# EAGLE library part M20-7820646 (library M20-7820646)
M20: 6 Pos Receptacle SIL Straight 3mm THT Connector 8.5mm high Tin Source: Datasheet
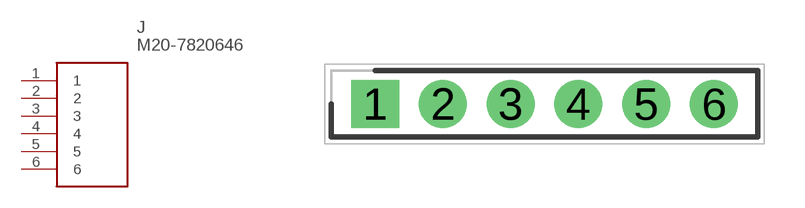
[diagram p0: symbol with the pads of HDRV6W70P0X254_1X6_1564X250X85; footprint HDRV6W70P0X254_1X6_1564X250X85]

Designator prefix J

## M20-7820646 (Description: M20: 6 Pos Receptacle SIL Straight 3mm THT Connector 8.5mm high Tin; Height: 8.5mm; Manufacturer_Name: Harwin; Manufacturer_Part_Number: M20-7820646; Mouser_Part_Number: 855-M20-7820646; Mouser_Price-Stock: https://www.mouser.co.uk/ProductDetail/Harwin/M20-7820646?qs=WS5Jv%252B%252Bx1qWZs4rbTjPGWw%3D%3D)  [HDRV6W70P0X254_1X6_1564X250X85]
1  1
2  2
3  3
4  4
5  5
6  6

## Footprint HDRV6W70P0X254_1X6_1564X250X85 (pad centres in mm)
6pin header1
drill 1.2 pad 1.8 square: 1 0,0
drill 1.2 pad 1.8: 2 2.54,0; 3 5.08,0; 4 7.62,0; 5 10.16,0; 6 12.7,0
